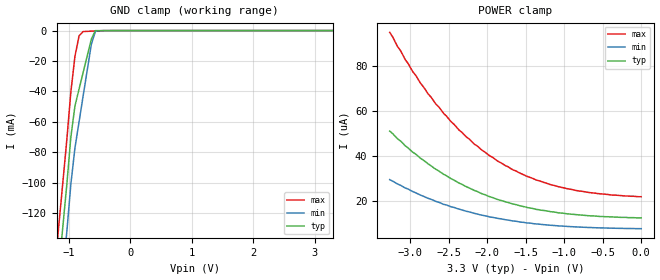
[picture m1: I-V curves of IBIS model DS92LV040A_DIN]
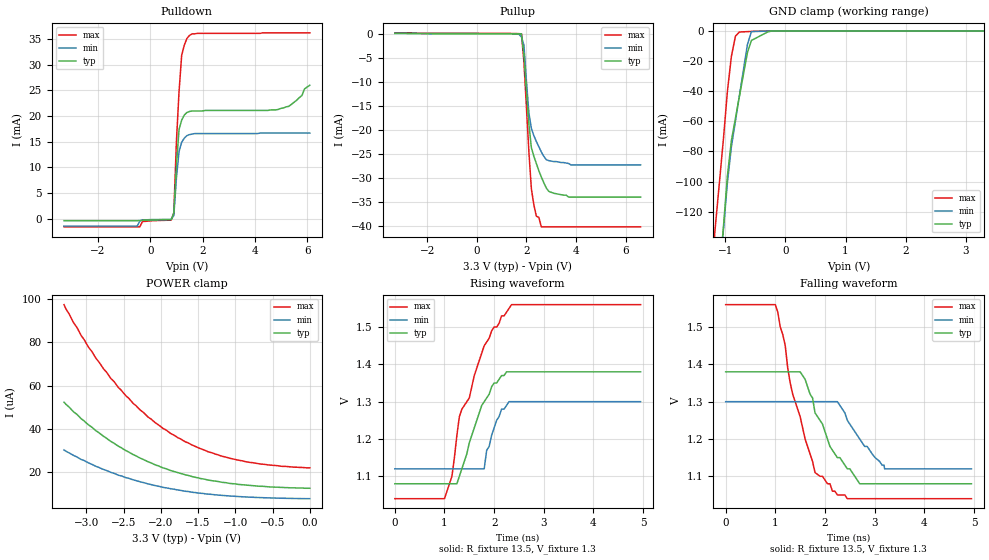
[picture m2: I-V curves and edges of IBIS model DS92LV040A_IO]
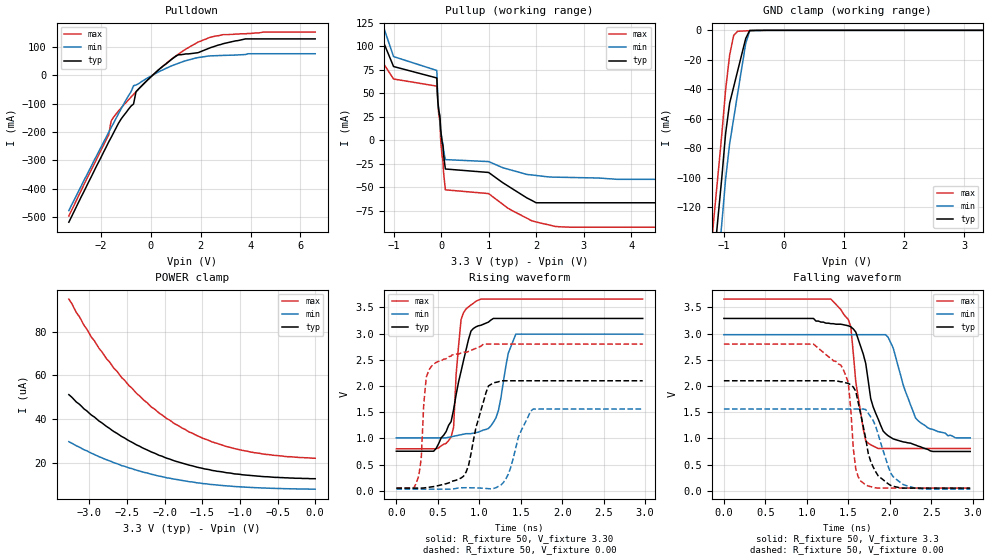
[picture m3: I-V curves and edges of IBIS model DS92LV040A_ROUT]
|   National Semiconductor Corporation
|   IBIS Model of DS92LV040A
|   4 Channel Bus LVDS Transceiver
|   44 Lead LLP Package
[IBIS Ver]   3.2
[Comment Char]   |_char
[File name]   ds92lv040a.ibs
[File Rev]   2.1
[Date]   05/2/02
[Source]
SPICE to IBIS Translation
[Notes]
Created by Tim Coyle
adjusted IOM and IOP rise fall tables for monotonicity--milt
[Disclaimer]
(C) Copyright National Semiconductor Corporation 2002
   All rights reserved
   National Semiconductor Corporation hereby grants
the user of this IBIS model a non-exclusive, nontransferable
license to use this IBIS model under the following terms.
Before using this IBIS model, the user should read this
license.  If the user does not accept these terms,  the
IBIS model should be returned to National within 30 days.
   The user is granted this license only to use the
IBIS model and is not granted rights to sell, load, rent,
lease or license the IBIS model in whole or in part, or in
modified form to anyone other than user. User may modify
the IBIS model to suit its specific applications but rights
to derivative works and such modifications shall belong to
National.
   This IBIS model is provided on an "AS IS" basis and
National makes absolutely no warranty with respect to the
information contained herein.NATIONAL DISCLAIMS AND CUSTOMER
WAIVES ALL WARRANTIES, EXPRESS OR IMPLIED, INCLUDING
WARRANTIES OF MERCHANTABILITY OR FITNESS FOR A PARTICULAR
PURPOSE. The entire risk as to quality and performance is
with the Customer. ACCORDINGLY, IN NO EVENT SHALL THE
COMPANY BE LIABLE FOR ANY DAMAGES, WHETHER IN CONTRACT OR
TORT,INCLUDING ANY LOST PROFITS OR OTHER INCIDENTAL,
CONSEQUENTIAL, EXEMPLARY, OR PUNITIVE DAMAGES ARISING OUT
OF THE USE OR APPLICATION OF THE IBIS model provided in
this package.Further, National reserves the right to make
changes without notice to any product herein to improve
reliability, function, or design. National does not convey
any license under patent rights or any other intellectual
property rights, including those of third parties.
   National is not obligated to provide maintenance or support
for the licensed IBIS model.
Contact National at ATTN:INTERFACE APPLICATIONS/IBIS MODELS.
5 Foden Road, M/S 03-03, South Porltand, ME 04106
(207) 541-8203
[Copyright]
(c) Copyright 2002 National Semiconductor Corp.
[Component]   DS92LV040A
Si_location Pin
Timing_location Pin
[Manufacturer]   National Semiconductor Corp.
[Package]
|   TYP   MIN   MAX
R_pkg   50.0m   NA   NA
L_pkg   1.88nH   NA   NA
C_pkg   0.306pF   NA   NA
[Pin]   signal_name  model_name   R_pin   L_pin   C_pin
1   NC   NC   50.0m   2.11433n   0.27505p
2   NC   NC   50.0m   2.01554n   0.33960p
3   VCC   POWER   50.0m   1.94357n   0.32802p
4   GND   GND   50.0m   1.89274n   0.32012p
5   RE2*   DS92LV040A_CONTROL 50.0m   1.83759n   0.31097p
6   VCC   POWER   50.0m   1.79220n   0.30663p
7   AVCC   POWER   50.0m   1.74406n   0.29967p
8   DE2   DS92LV040A_CONTROL 50.0m   1.74394n   0.31941p
9   AGND   GND   50.0m   1.74394n   0.31941p
10   VCC   POWER   50.0m   1.74406n   0.29967p
11   NC   NC   50.0m   1.79220n   0.30663p
12   NC   NC   50.0m   1.83759n   0.31097p
13   DO4-_RIN4-   DS92LV040A_IO   50.0m   1.89274n   0.32012p
14   DO4+_RIN4+   DS92LV040A_IO   50.0m   1.94357n   0.32802p
15   DO3-_RIN3-   DS92LV040A_IO   50.0m   2.01554n   0.33960p
16   DO3+_RIN3+   DS92LV040A_IO   50.0m   2.11433n   0.27505p
17   AGND   GND   50.0m   2.11433n   0.27505p
18   DO2-_RIN2-   DS92LV040A_IO   50.0m   2.01554n   0.33960p
19   DO2+_RIN2+   DS92LV040A_IO   50.0m   1.94357n   0.32802p
20   DO1-_RIN1-   DS92LV040A_IO   50.0m   1.89274n   0.32012p
21   DO1+_RIN1+   DS92LV040A_IO   50.0m   1.83759n   0.31097p
22   AVCC   POWER   50.0m   1.79220n   0.30663p
23   NC   NC   50.0m   1.74406n   0.29967p
24   NC   NC   50.0m   1.74394n   0.31941p
25   AGND   GND   50.0m   1.74394n   0.31941p
26   DE1   DS92LV040A_CONTROL 50.0m   1.74406n   0.29967p
27   AVCC   POWER   50.0m   1.79220n   0.30663p
28   GND   GND   50.0m   1.83759n   0.31097p
29   RE1*   DS92LV040A_CONTROL 50.0m   1.89274n   0.32012p
30   VCC   POWER   50.0m   1.94357n   0.32802p
31   GND   GND   50.0m   2.01554n   0.33960p
32   NC   NC   50.0m   2.11433n   0.27505p
33   NC   NC   50.0m   2.11433n   0.27505p
34   NC   NC   50.0m   2.01554n   0.33960p
35   DIN1   DS92LV040A_DIN   50.0m   1.94357n   0.32802p
36   RO1   DS92LV040A_ROUT   50.0m   1.89274n   0.32012p
37   DIN2   DS92LV040A_DIN   50.0m   1.83759n   0.31097p
38   RO2   DS92LV040A_ROUT   50.0m   1.89274n   0.32012p
39   GND   GND   50.0m   1.74406n   0.29967p
40   DIN3   DS92LV040A_DIN   50.0m   1.74394n   0.31941p
41   RO3   DS92LV040A_ROUT   50.0m   1.89274n   0.32012p
42   DIN4   DS92LV040A_DIN   50.0m   1.74406n   0.29967p
43   RO4   DS92LV040A_ROUT   50.0m   1.89274n   0.32012p
44   NC   NC   50.0m   1.83759n   0.31097p
[Diff Pin] inv_pin   vdiff   tdelay_typ   tdelay_min   tdelay_max
| The '+' pin is Diff_pin and the '-' pin is the inv_pin
| Receiver Vth = +/-100mV
14   13   0.1   0   0   0
16   15   0.1   0   0   0
19   18   0.1   0   0   0
21   20   0.1   0   0   0
| Models and submodels in the file (4): DS92LV040A_DIN (Input), DS92LV040A_IO (I/O), DS92LV040A_ROUT (Output), DS92LV040A_CONTROL (Input)
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[Model]   DS92LV040A_DIN
Model_type Input
Vinh=2.0
Vinl=0.8
C_comp   3.834p   NA   NA
[Temperature Range] 25   85   -40
[Voltage Range]   3.3   3.00   3.60
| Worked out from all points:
|   GND clamp passes 1 mA (typ) near -0.58 V on its own axis
[GND Clamp]
|V(groundclamp)   I(typ)   I(min)   I(max)
-3.3V     -1.29A     -1.28A     -1.31A
-1.17V    -161mA     -192mA     -131mA
-1.1V     -130mA     -161mA     -101mA
-1.03V    -100mA     -131mA     -70.6mA
-967mV    -70mA      -101mA     -40.4mA
-900mV    -49.4mA    -76.9mA    -16.8mA
-833mV    -38.4mA    -59.9mA    -3.44mA
-767mV    -27.5mA    -42.9mA    -643uA
-633mV    -5.52mA    -8.94mA    -387uA
-567mV    -32.1uA    -395uA     -259uA
3.3V      456pA      883pA      215pA
[POWER Clamp]
|Vtable   I(typ)   I(min)   I(max)
-3.27V    51.2uA     29.6uA     95.1uA
-3.17V    47.8uA     27.7uA     88.9uA
-2.97V    41.8uA     24.3uA     77.6uA
-2.77V    36.6uA     21.3uA     67.7uA
-2.57V    32uA       18.6uA     59.1uA
-2.37V    28.1uA     16.5uA     51.7uA
-2.17V    24.8uA     14.6uA     45.4uA
-1.87V    20.8uA     12.4uA     37.9uA
-1.5V     17.4uA     10.4uA     31.3uA
-1.07V    14.8uA     9.01uA     26.4uA
-666mV    13.5uA     8.3uA      23.8uA
0V        12.6uA     7.79uA     22uA
[Model]   DS92LV040A_IO
Model_type I/O
Polarity Non-Inverting
Vref=1.30
Vmeas=1.25
Rref=13.5   | 27 Ohms Across Outputs OUTP and OUTM
Cref=5p
Vinl = -0.1
Vinh =  0.1
C_comp   3.108p   NA   NA
[Temperature Range] 25   85   -40
[Voltage Range]   3.3   3.00   3.60
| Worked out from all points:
|   slope of the pulldown table from 0 to 0.495 V, typ, clamps not added: 11.3 kohm
|   GND clamp passes 1 mA (typ) near -0.31 V on its own axis
|   falling waveform, R_fixture 13.5, V_fixture 1.3: 20-80 % time 650ps typ, 559ps min, 550ps max; typ from 1.38 V to 1.08 V
|   rising waveform, R_fixture 13.5, V_fixture 1.3: 20-80 % time 500ps typ, 274ps min, 636ps max; typ from 1.08 V to 1.38 V
[Pullup]
|Vtable   I(typ)   I(min)   I(max)
-3.3V     246uA      198uA      325uA
1.6V      117uA      115uA      172uA
1.8V      103uA      -541uA     120uA
1.9V      -4.37mA    -2.21mA    -5.79mA
2.1V      -18.7mA    -16.4mA    -24.5mA
2.2V      -23.6mA    -19.6mA    -32.2mA
2.4V      -26.9mA    -22.3mA    -37.9mA
2.5V      -28.4mA    -23.4mA    -38.1mA
2.6V      -29.7mA    -24.5mA    -40.1mA
2.9V      -32.7mA    -26.3mA    -40.1mA
3.7V      -33.9mA    -26.9mA    -40.1mA
6.6V      -33.9mA    -27.2mA    -40.1mA
[Pulldown]
|V(pulldown)   I(typ)   I(min)   I(max)
-3.3V     -351uA     -1.4mA     -1.55mA
-500mV    -351uA     -1.4mA     -1.55mA
-400mV    -322uA     -431uA     -1.55mA
800mV     -164uA     -95.3uA    -250uA
900mV     1.14mA     641uA      1.2mA
1V        10.4mA     7.96mA     15.1mA
1.1V      17.4mA     13.1mA     24.8mA
1.2V      19.2mA     14.9mA     31.8mA
1.5V      20.9mA     16.4mA     35.7mA
4.9V      21.3mA     16.7mA     36.2mA
5.3V      21.9mA     16.7mA     36.2mA
6.1V      26mA       16.7mA     36.2mA
[GND Clamp]
|V(groundclamp)   I(typ)   I(min)   I(max)
-3.3V     -1.36A     -1.28A     -1.31A
-1.17V    -195mA     -192mA     -131mA
-1.1V     -162mA     -161mA     -101mA
-1.03V    -129mA     -131mA     -70.6mA
-967mV    -96.5mA    -101mA     -40.4mA
-900mV    -72.8mA    -76.9mA    -16.8mA
-833mV    -58.1mA    -59.9mA    -3.44mA
-767mV    -43.5mA    -42.9mA    -643uA
-633mV    -14.3mA    -8.94mA    -387uA
-567mV    -6.25mA    -395uA     -259uA
-233mV    -5.33uA    -194nA     -1.26uA
3.3V      984pA      883pA      215pA
[POWER Clamp]
|Vtable   I(typ)   I(min)   I(max)
-3.3V     52.3uA     30.3uA     97.3uA
-3.17V    47.8uA     27.7uA     88.9uA
-2.97V    41.8uA     24.3uA     77.6uA
-2.67V    34.2uA     19.9uA     63.2uA
-2.47V    30uA       17.5uA     55.3uA
-2.27V    26.4uA     15.5uA     48.5uA
-2.07V    23.3uA     13.8uA     42.7uA
-1.87V    20.8uA     12.4uA     37.9uA
-1.5V     17.4uA     10.4uA     31.3uA
-1.07V    14.8uA     9.01uA     26.4uA
-666mV    13.5uA     8.3uA      23.8uA
0V        12.6uA     7.79uA     22uA
|IO
[Ramp]
dV/dt_r   180mV/.500ns   108mV/.750ns   312mV/.400ns
dV/dt_f   180mv/.650ns   108mv/.750ns   312mv/.400ns
R_load=13.5
|IO
[Falling Waveform]
R_fixture=13.5
V_fixture=1.3
V_fixture_min=1.3
V_fixture_max=1.3
0s        1.38V      1.3V       1.56V
1ns       1.38V      1.3V       1.56V
1.2ns     1.38V      1.3V       1.45V
1.3ns     1.38V      1.3V       1.35V
1.5ns     1.38V      1.3V       1.26V
1.8ns     1.27V      1.3V       1.11V
2.15ns    1.17V      1.3V       1.06V
2.7ns     1.08V      1.2V       1.04V
3.2ns     1.08V      1.12V      1.04V
4.95ns    1.08V      1.12V      1.04V
|IO
[Rising Waveform]
R_fixture=13.5
V_fixture=1.3
V_fixture_min=1.3
V_fixture_max=1.3
0s        1.08V      1.12V      1.04V
1ns       1.08V      1.12V      1.04V
1.15ns    1.08V      1.12V      1.1V
1.25ns    1.08V      1.12V      1.21V
1.3ns     1.1V       1.12V      1.26V
1.5ns     1.19V      1.12V      1.31V
1.8ns     1.3V       1.12V      1.45V
2.05ns    1.35V      1.25V      1.5V
2.35ns    1.38V      1.3V       1.56V
4.95ns    1.38V      1.3V       1.56V
[Model]   DS92LV040A_ROUT
Model_type Output
Polarity Non-Inverting
Vref=0.0
Vmeas=1.65
Cref=15p
C_comp   4.097p   NA   NA
[Temperature Range] 25   85   -40
[Voltage Range]   3.3   3.00   3.60
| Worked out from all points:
|   slope of the pulldown table from 0 to 0.495 V, typ, clamps not added: 12.9 ohm
|   slope of the pullup table from 0 to 0.495 V, typ, clamps not added: 12.4 ohm
|   GND clamp passes 1 mA (typ) near -0.58 V on its own axis
|   falling waveform, R_fixture 50, V_fixture 3.3: 20-80 % time 245ps typ, 241ps min, 128ps max; typ from 3.29 V to 0.75 V
|   rising waveform, R_fixture 50, V_fixture 3.30: 20-80 % time 219ps typ, 142ps min, 74.2ps max; typ from 0.755 V to 3.29 V
|   falling waveform, R_fixture 50, V_fixture 0.00: 20-80 % time 179ps typ, 188ps min, 120ps max; typ from 2.1 V to 0.05 V
|   rising waveform, R_fixture 50, V_fixture 0.00: 20-80 % time 183ps typ, 184ps min, 80.6ps max; typ from 0.05 V to 2.1 V
[Pullup]
|Vtable   I(typ)   I(min)   I(max)
-3.3V     539mA      529mA      495mA
-1.4V     137mA      151mA      159mA
-1.3V     120mA      135mA      89.1mA
-1.2V     103mA      119mA      80.9mA
-1V       78.5mA     89.1mA     65.2mA
-90mV     66.3mA     74.3mA     57.6mA
-70mV     42mA       44.5mA     42.5mA
-10mV     12mA       10.6mA     920uA
90mV      -30.7mA    -20.7mA    -52.9mA
1V        -34.4mA    -22.8mA    -56.9mA
2V        -66.7mA    -37.6mA    -87.2mA
6.6V      -66.7mA    -41.7mA    -92.7mA
[Pulldown]
|V(pulldown)   I(typ)   I(min)   I(max)
-3.3V     -518mA     -477mA     -496mA
-1.7V     -235mA     -201mA     -210mA
-1.6V     -219mA     -184mA     -161mA
-1.2V     -154mA     -118mA     -115mA
-700mV    -101mA     -36.2mA    -66.9mA
-600mV    -57.4mA    -33.7mA    -57.4mA
900mV     61.5mA     36.3mA     62.5mA
1.1V      72.9mA     42.8mA     74.9mA
1.9V      80.4mA     63mA       118mA
2.9V      112mA      70.7mA     144mA
3.8V      129mA      73.8mA     147mA
6.6V      129mA      76.6mA     153mA
[GND Clamp]
|V(groundclamp)   I(typ)   I(min)   I(max)
-3.3V     -1.29A     -1.28A     -1.31A
-1.17V    -161mA     -192mA     -131mA
-1.1V     -130mA     -161mA     -101mA
-1.03V    -100mA     -131mA     -70.6mA
-967mV    -70mA      -101mA     -40.4mA
-900mV    -49.4mA    -76.9mA    -16.8mA
-833mV    -38.4mA    -59.9mA    -3.44mA
-767mV    -27.5mA    -42.9mA    -643uA
-633mV    -5.52mA    -8.94mA    -387uA
-567mV    -32.1uA    -395uA     -259uA
3.3V      456pA      883pA      215pA
[POWER Clamp]
|Vtable   I(typ)   I(min)   I(max)
-3.27V    51.2uA     29.6uA     95.1uA
-3.17V    47.8uA     27.7uA     88.9uA
-2.97V    41.8uA     24.3uA     77.6uA
-2.77V    36.6uA     21.3uA     67.7uA
-2.57V    32uA       18.6uA     59.1uA
-2.37V    28.1uA     16.5uA     51.7uA
-2.17V    24.8uA     14.6uA     45.4uA
-1.87V    20.8uA     12.4uA     37.9uA
-1.5V     17.4uA     10.4uA     31.3uA
-1.07V    14.8uA     9.01uA     26.4uA
-666mV    13.5uA     8.3uA      23.8uA
0V        12.6uA     7.79uA     22uA
[Ramp]
dV/dt_r   2.0V/1ns   1.8V/2ns   2.2V/.8ns
dV/dt_f   2.0V/1ns   1.8V/2ns   2.2V/.8ns
R_load=50
[Falling Waveform]
R_fixture=50
V_fixture=3.3
V_fixture_min=3.00
V_fixture_max=3.60
0s        3.29V      2.98V      3.66V
1.29ns    3.19V      2.98V      3.66V
1.53ns    3.13V      2.98V      3.13V
1.59ns    3.03V      2.98V      2.08V
1.71ns    2.43V      2.98V      950mV
1.77ns    1.76V      2.98V      877mV
1.95ns    1.09V      2.98V      806mV
2.04ns    991mV      2.73V      806mV
2.31ns    873mV      1.39V      806mV
2.97ns    750mV      1.01V      806mV
[Rising Waveform]
R_fixture=50
V_fixture=3.30
V_fixture_min=3.00
V_fixture_max=3.60
0s        755mV      1.01V      801mV
450ps     755mV      1.01V      801mV
660ps     1.32V      1.03V      1.03V
690ps     1.55V      1.04V      1.21V
720ps     1.83V      1.05V      2.21V
780ps     2.28V      1.07V      3.27V
960ps     3.13V      1.11V      3.62V
1.2ns     3.29V      1.39V      3.66V
1.44ns    3.29V      2.99V      3.66V
2.97ns    3.29V      2.99V      3.66V
[Falling Waveform]
R_fixture=50
V_fixture=0.00
V_fixture_min=0.00
V_fixture_max=0.00
0s        2.1V       1.56V      2.8V
1.08ns    2.1V       1.56V      2.8V
1.41ns    2.08V      1.56V      2.4V
1.5ns     2.05V      1.56V      2.06V
1.59ns    1.9V       1.56V      415mV
1.71ns    996mV      1.55V      111mV
1.86ns    285mV      1.08V      50.7mV
2.01ns    102mV      339mV      50.7mV
2.13ns    50.4mV     155mV      50.7mV
2.97ns    50.4mV     30mV       50.7mV
[Rising Waveform]
R_fixture=50
V_fixture=0.00
V_fixture_min=0.00
V_fixture_max=0.00
0s        50.3mV     30.2mV     50.5mV
270ps     50.3mV     30.2mV     284mV
300ps     50.3mV     30.2mV     615mV
360ps     59.3mV     30.2mV     2.16V
480ps     88.6mV     30.2mV     2.45V
840ps     355mV      58mV       2.64V
1.17ns    2.06V      41.8mV     2.8V
1.35ns    2.1V       317mV      2.8V
1.65ns    2.1V       1.56V      2.8V
2.97ns    2.1V       1.56V      2.8V
